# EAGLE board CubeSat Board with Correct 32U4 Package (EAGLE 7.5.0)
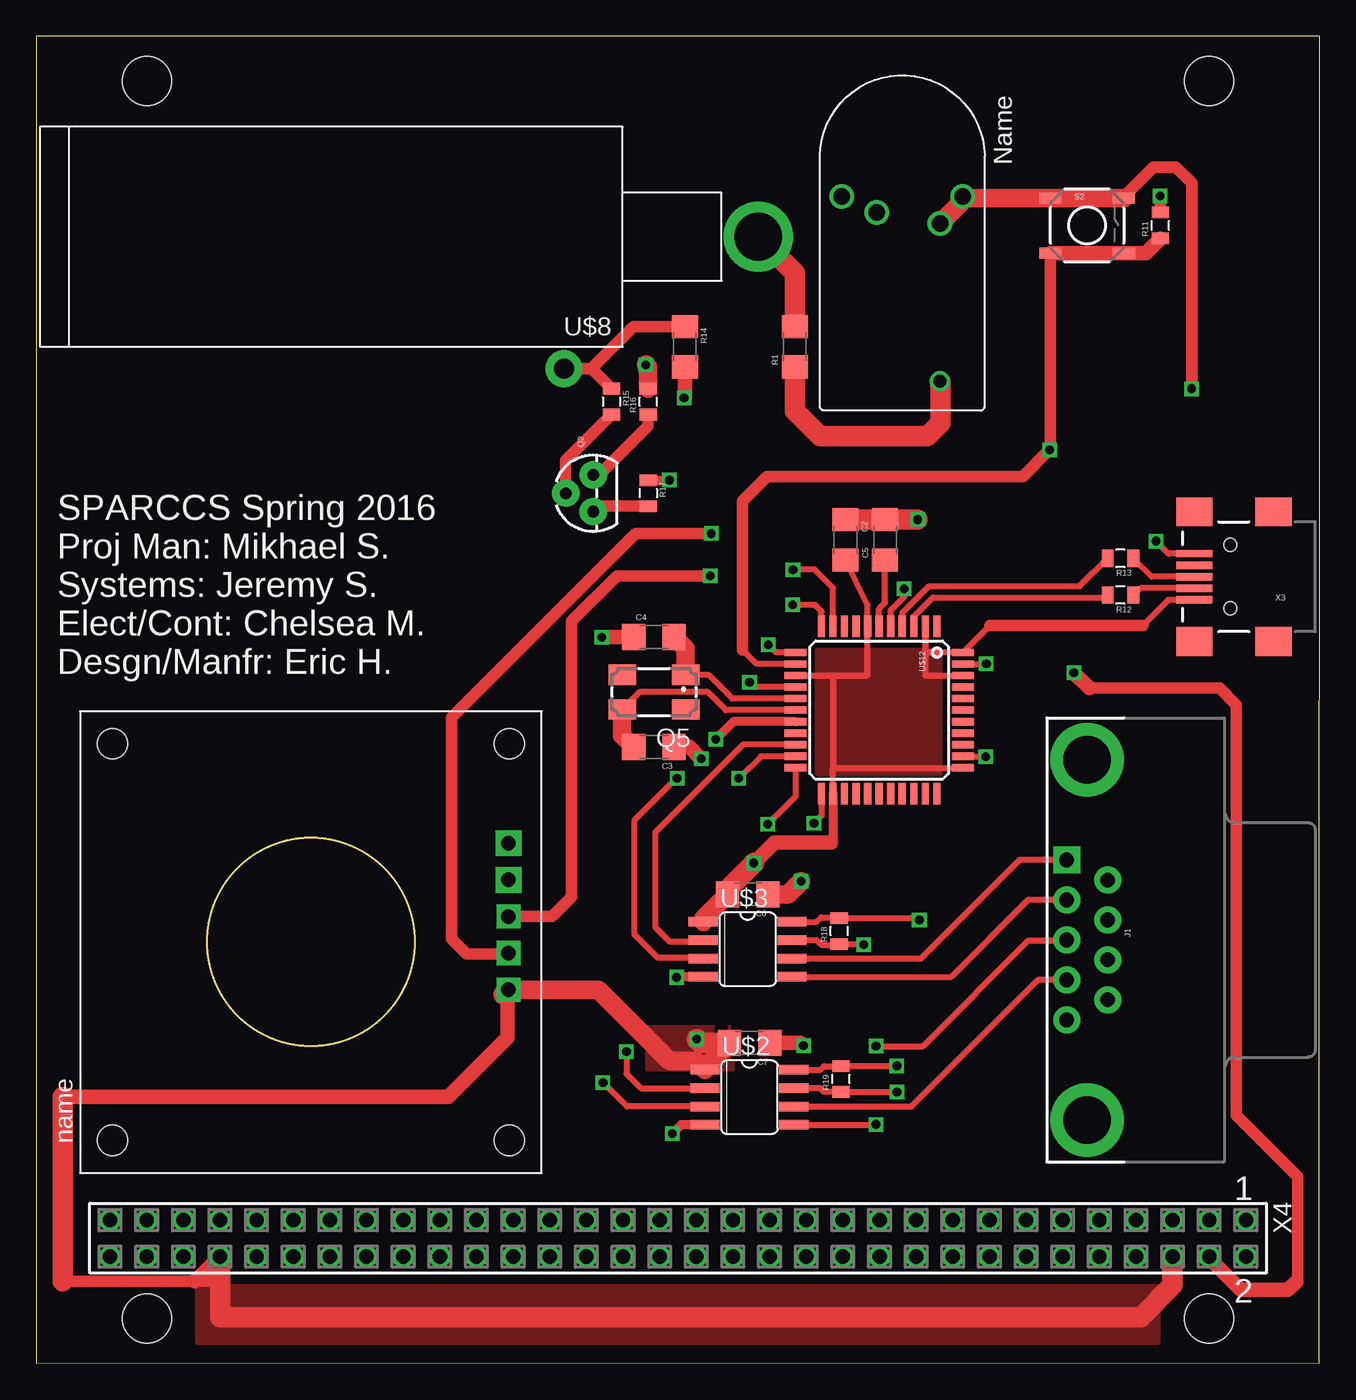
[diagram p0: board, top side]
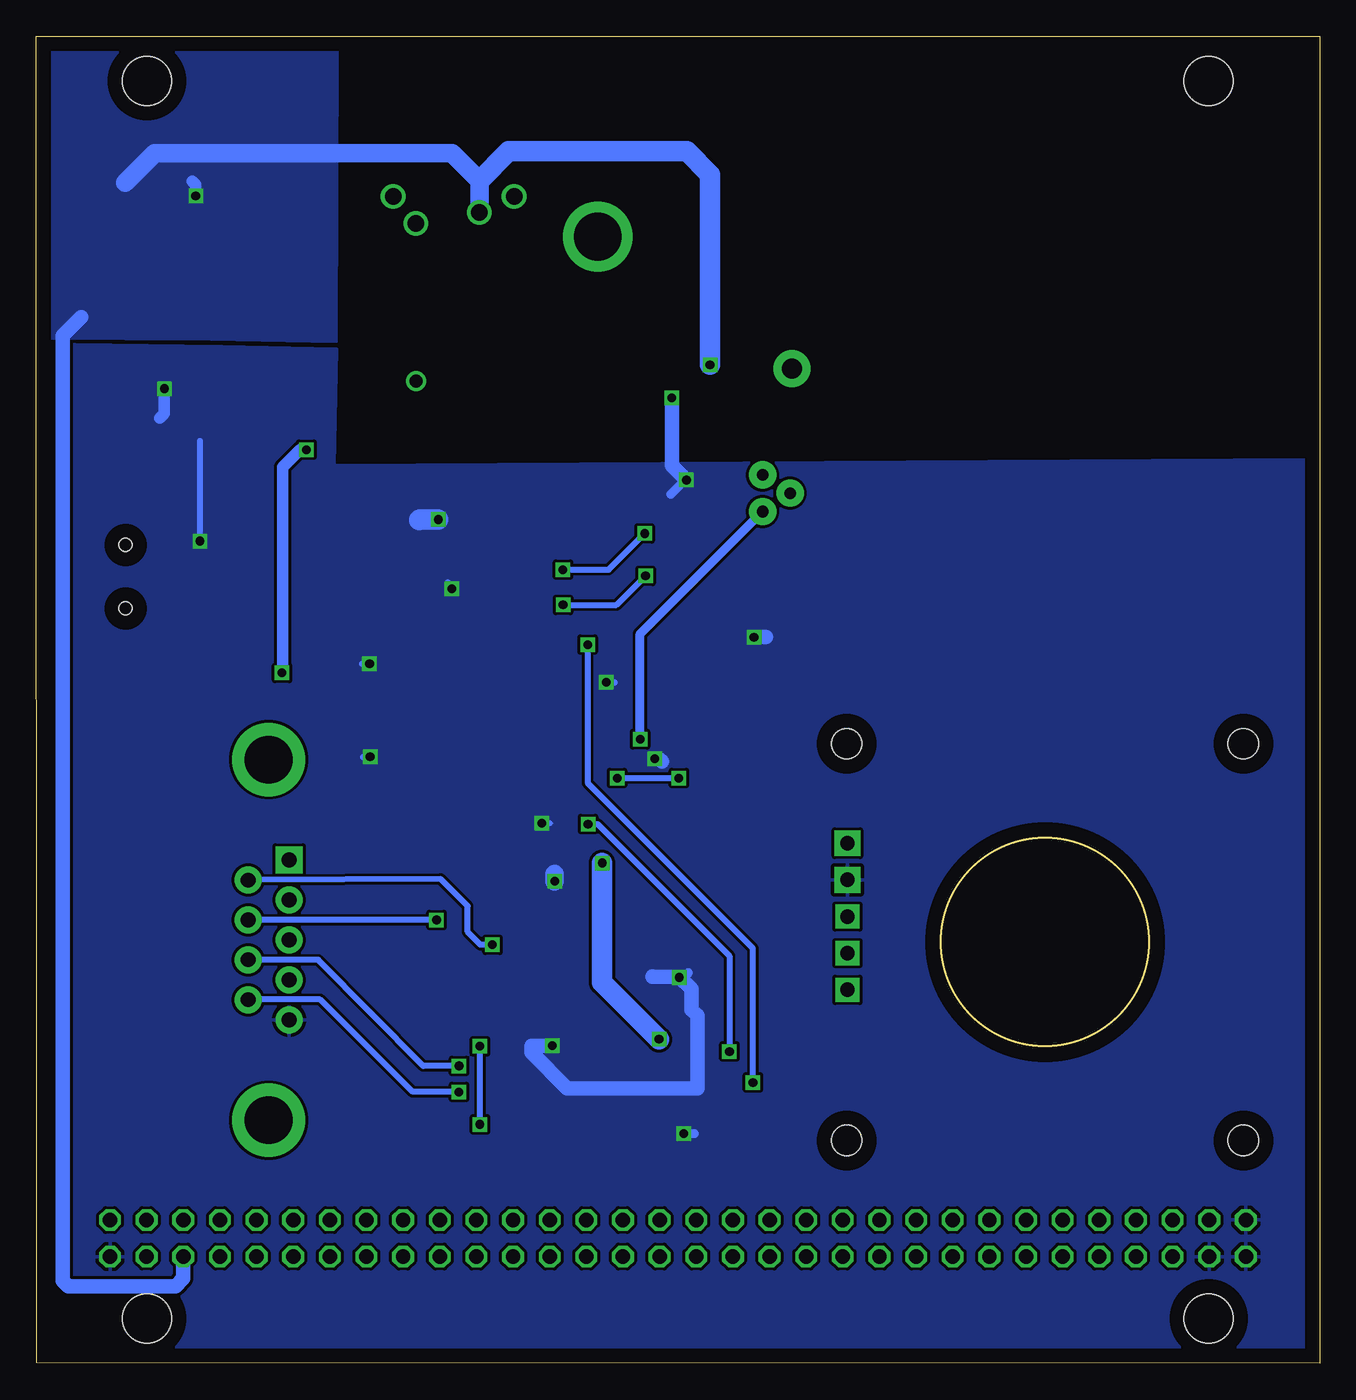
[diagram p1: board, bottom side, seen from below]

Size 89 x 92.02 mm. Coordinates in mm from the lower left corner, seen from the top.
Outline: 0,0 88.95,0.03 89,92.02 0,92.01 0,0
Copper layers (1*16): Top 0.035mm / dielectric 1.5mm / Bottom 0.035mm
Design rules "default": minimum track width 10mil, minimum drill 24mil, track to track 8mil, track to pad 8mil, pad to pad 8mil, via to via 8mil, smd to smd 8mil, copper to edge 40mil, drill to drill 8mil, minimum pad ring 10mil, minimum via ring 8mil, stop-mask expansion 4mil, vias tented up to drill 0mil, thermal gap 10mil
Holes 3.4 mm at 7.7,3.1 81.3,3.1 81.3,88.9 7.7,88.9

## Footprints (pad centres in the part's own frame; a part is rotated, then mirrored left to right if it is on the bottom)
1206 = smd 1.6 x 1.8: 1 -1.4,0; 2 1.4,0
ASERIES = drill 1.143: (+)IN -2.032,-1.778; (-)IN -3.15,4.191; CNTRL -3.15,-4.191; HVRTN -1.27,2.616 | drill 0.889: HVOUT 9.652,2.616
DB9 = drill 1.016 pad 1.88 square: 1 -5.54,-1.42 | drill 1.016 pad 1.88: 2 -2.77,-1.42; 3 0,-1.42; 4 2.77,-1.42; 5 5.54,-1.42; 6 -4.15,1.42; 7 -1.38,1.42; 8 1.38,1.42; 9 4.15,1.42 | drill 3.302 pad 5.08: G1 -12.5,0; G2 12.5,0
TO-92 = drill 0.813 pad 1.88: 1 -1.27,0; 2 0,1.905; 3 1.27,0
CTS406 = smd 1.9 x 1.4: 1 -2.2,-1.2; 2 2.2,-1.2; 3 2.2,1.2; 4 -2.2,1.2
0805 = smd 0.8 x 1.2: 1 -0.9,0; 2 0.9,0
TACTILE_SWITCH_SMD = smd 1.524 x 0.762: 1 -2.54,1.905; 2 2.54,1.905; 3 -2.54,-1.905; 4 2.54,-1.905
SO-08 = smd 0.66 x 2.032: 1 -1.905,-3.073; 2 -0.635,-3.073; 3 0.635,-3.073; 4 1.905,-3.073; 5 1.905,3.073; 6 0.635,3.073; 7 -0.635,3.073; 8 -1.905,3.073
GEIGER_TUBE = drill 1.4 pad 2.54: GND 13.462,9.144 | drill 3.302 pad 4.826: VCC 0,0
UCAM-II = drill 1 pad 1.676 square: 5V -3.31,-13.7; RX 1.77,-13.7; TX -0.77,-13.7 | drill 1 pad 1.778 square: GND 4.31,-13.7; RES 6.85,-13.7 | hole 2.1: -13.75,-13.75; 13.75,-13.75; 13.75,13.75; -13.75,13.75
SPARKFUN-DIGITALIC_TQFP44 = smd 1.5 x 0.5: 1 -5.8,4; 2 -5.8,3.2; 3 -5.8,2.4; 4 -5.8,1.6; 5 -5.8,0.8; 6 -5.8,0; 7 -5.8,-0.8; 8 -5.8,-1.6; 9 -5.8,-2.4; 10 -5.8,-3.2; 11 -5.8,-4; 23 5.8,-4; 24 5.8,-3.2; 25 5.8,-2.4; 26 5.8,-1.6; 27 5.8,-0.8; 28 5.8,0; 29 5.8,0.8; 30 5.8,1.6; 31 5.8,2.4; 32 5.8,3.2; 33 5.8,4 | smd 0.5 x 1.5: 12 -4,-5.8; 13 -3.2,-5.8; 14 -2.4,-5.8; 15 -1.6,-5.8; 16 -0.8,-5.8; 17 0,-5.8; 18 0.8,-5.8; 19 1.6,-5.8; 20 2.4,-5.8; 21 3.2,-5.8; 22 4,-5.8; 34 4,5.8; 35 3.2,5.8; 36 2.4,5.8; 37 1.6,5.8; 38 0.8,5.8; 39 0,5.8; 40 -0.8,5.8; 41 -1.6,5.8; 42 -2.4,5.8; 43 -3.2,5.8; 44 -4,5.8
USB-MINIB = smd 2.5 x 0.5: D+ 2.5,0; D- 2.5,0.8; GND 2.5,-1.6; ID 2.5,-0.8; VBUS 2.5,1.6 | smd 2.5 x 2: MTN1 -3,4.5; MTN2 2.5,4.5; MTN3 -3,-4.5; MTN4 2.5,-4.5 | hole 0.9: 0,2.2; 0,-2.2
SSW-132-02-S-D = drill 1 pad 1.5 octagon: 1 -39.37,-1.27; 2 -39.37,1.27; 3 -36.83,-1.27; 4 -36.83,1.27; 5 -34.29,-1.27; 6 -34.29,1.27; 7 -31.75,-1.27; 8 -31.75,1.27; 9 -29.21,-1.27; 10 -29.21,1.27; 11 -26.67,-1.27; 12 -26.67,1.27; 13 -24.13,-1.27; 14 -24.13,1.27; 15 -21.59,-1.27; 16 -21.59,1.27; 17 -19.05,-1.27; 18 -19.05,1.27; 19 -16.51,-1.27; 20 -16.51,1.27; 21 -13.97,-1.27; 22 -13.97,1.27; 23 -11.43,-1.27; 24 -11.43,1.27; 25 -8.89,-1.27; 26 -8.89,1.27; 27 -6.35,-1.27; 28 -6.35,1.27; 29 -3.81,-1.27; 30 -3.81,1.27; 31 -1.27,-1.27; 32 -1.27,1.27; 33 1.27,-1.27; 34 1.27,1.27; 35 3.81,-1.27; 36 3.81,1.27; 37 6.35,-1.27; 38 6.35,1.27; 39 8.89,-1.27; 40 8.89,1.27; 41 11.43,-1.27; 42 11.43,1.27; 43 13.97,-1.27; 44 13.97,1.27; 45 16.51,-1.27; 46 16.51,1.27; 47 19.05,-1.27; 48 19.05,1.27; 49 21.59,-1.27; 50 21.59,1.27; 51 24.13,-1.27; 52 24.13,1.27; 53 26.67,-1.27; 54 26.67,1.27; 55 29.21,-1.27; 56 29.21,1.27; 57 31.75,-1.27; 58 31.75,1.27; 59 34.29,-1.27; 60 34.29,1.27; 61 36.83,-1.27; 62 36.83,1.27; 63 39.37,-1.27; 64 39.37,1.27

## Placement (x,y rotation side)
C2  0.1uF  [1206]  56.11,57.09 270 top
C3  18pF  [1206]  42.84,42.73 180 top
C4  18pF  [1206]  42.84,50.35 0 top
C5  1uF  [1206]  58.85,57.09 90 top
C6  0.1uF  [1206]  49.33,32.52 180 top
C7  0.1uF  [1206]  49.47,22.23 180 top
DC-HVDC  A06  [ASERIES]  60.05,77.75 270 top
J1  DB9 Connector  [DB9]  72.87,29.36 270 top
Q2  MPSA18  [TO-92]  38.62,60.33 90 top
Q5  16MHz  [CTS406]  42.84,46.54 180 top
R1  10M  [1206]  52.59,70.48 90 top
R11  10k  [0805]  77.94,78.89 90 top
R12  22  [0805]  75.17,53.27 180 top
R13  22  [0805]  75.17,55.8 180 top
R14  1M  [1206]  44.98,70.48 270 top
R15  10M  [0805]  39.9,66.67 270 top
R16  15k  [0805]  42.44,66.67 90 top
R17  1M  [0805]  42.44,60.33 270 top
R18  120  [0805]  55.68,29.98 90 top
R19  120  [0805]  55.8,19.73 90 top
S2  Reset  [TACTILE_SWITCH_SMD]  72.86,78.89 0 top
U$2  MAX488  [SO-08]  49.45,18.45 270 top
U$3  MAX488  [SO-08]  49.33,28.71 270 top
U$8  GEIGER_TUBELND712  [GEIGER_TUBE]  50.05,78.11 180 top
U$9  UCAM-II  [UCAM-II]  19.05,29.21 90 top
U$12  ATMEGA32U4TQFP  [SPARKFUN-DIGITALIC_TQFP44]  58.45,45.29 270 top
X3  USBSMD  [USB-MINIB]  82.78,54.53 180 top
X4  SSW-132-02-S-D  [SSW-132-02-S-D]  44.5,8.68 180 top

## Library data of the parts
C2-C7 = SparkFun-Passives
DC-HVDC = aseries
J1 = SparkFun-Connectors; PROD_ID: CONN-08194
Q2 R1 R11-R19 S2 U$8 X3 = SparkFun
Q5 = crystal; OC_FARNELL: unknown; OC_NEWARK: unknown
U$2 U$3 = max
U$9 = camera
U$12 = SparkFun-Retired; PROD_ID: IC-11161
X4 = con-samtec; MPN: SSW-132-02-S-D; OC_FARNELL: unknown; OC_NEWARK: 11P9837

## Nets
CTS+: J1.9 R19.1 U$2.7
CTS-: J1.8 R19.2 U$2.8
GND: C2.1 C3.1 C4.1 C5.2 C6.1 C7.1 DC-HVDC.(-)IN DC-HVDC.HVRTN J1.5 R14.2 R17.1 S2.1 S2.2 U$2.4 U$3.4 U$9.GND U$12.5 U$12.15 U$12.23 U$12.35 U$12.43 X3.GND X4.2 X4.62 X4.63 X4.64
MISO: U$9.RX U$12.11
MOSI: U$9.TX U$12.10
N$1: C3.2 Q5.3 U$12.17
N$2: R1.2 U$8.VCC
N$3: R14.1 R15.1 U$8.GND
N$4: DC-HVDC.HVOUT R1.1
N$5: Q2.2 R15.2
N$7: C4.2 Q5.1 U$12.16
N$8: Q2.3 R16.1
N$19: R12.1 X3.D-
N$21: R13.1 X3.D+
N$24: R12.2 U$12.3
N$25: R13.2 U$12.4
N$26: C5.1 U$12.6
OUT: Q2.1 R17.2 U$12.18
RST: R11.1 S2.3 S2.4 U$12.13 X4.4
RTS+: J1.4 U$2.6
RTS-: J1.3 U$2.5
RX: U$3.2 U$12.20
RX+: J1.7 R18.2 U$3.8
RX-: J1.6 R18.1 U$3.7
TX: U$3.3 U$12.21
TX+: J1.2 U$3.5
TX-: J1.1 U$3.6
VCC: C2.2 C6.2 C7.2 DC-HVDC.(+)IN R11.2 R16.2 U$2.1 U$3.1 U$9.5V U$12.2 U$12.7 U$12.14 U$12.24 U$12.34 U$12.42 U$12.44 X3.VBUS X4.6 X4.58
~CTS: U$2.2 U$12.22
~RTS: U$2.3 U$12.12

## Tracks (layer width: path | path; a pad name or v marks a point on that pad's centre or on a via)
CTS+  (via drill 0.6)
  Top 0.406: U$2.7 54.35,19.09 54.59,18.85 55.77,18.85 R19.1 59.34,18.82 v59.68,18.82
  Bottom 0.406: v59.68,18.82 62.88,18.83 69.31,25.23 74.27,25.23 J1.9
CTS-  (via drill 0.6)
  Top 0.406: U$2.8 54.37,20.36 54.62,20.61 55.78,20.61 R19.2 v59.67,20.62
  Bottom 0.406: v59.67,20.62 62.16,20.62 69.43,27.98 74.21,27.98 J1.8
GND  (via drill 0.6)
  Top 0.406: U$12.15 49.77,46.89 v49.45,47.21 | U$12.5 59.24,52.23 60.18,53.17 v60.18,53.7 | U$12.43 v65.87,48.49 v65.88,48.49 | U$12.35 65.81,42.09 v65.83,42.06 | U$12.23 54.45,37.98 v53.92,37.45 | X3.GND 78.5,56.13 v77.64,57.01
  Top 0.61: U$2.4 44.72,16.55 v44.1,15.94 | R17.1 43.9,61.23 v43.91,61.24 | U$3.4 44.45,26.8 v44.4,26.76
  Top 0.813: S2.2 75.39,80.89 77.44,82.94 79,82.94 80.11,81.84 v80.11,67.58
  Top 1.016: C3.1 45.29,42.73 v46.1,41.91 | C4.1 v39.23,50.35 | R14.2 44.98,66.99 v44.92,66.94 | C7.1 53.01,22.23 v53.2,22.03
  Top 1.27: C6.1 52.14,32.52 v53.04,33.42 | S2.2 S2.1 64.35,80.79 DC-HVDC.(-)IN 64.24,80.59 DC-HVDC.HVRTN
  Top 1.422: C2.1 C5.2 v61.1,58.49 v61.11,58.5
  Bottom 0.406: v49.45,47.21 49.05,47.21 49.04,47.22 48.91,47.22 48.9,47.2 48.88,47.22 | v60.18,53.7 60.18,53.88 60.47,54.16 | v65.88,48.49 66.29,48.49 66.3,48.48 66.3,48.49 66.42,48.49 66.42,48.5 | v65.83,42.06 66.31,42.06 66.33,42.04 | v53.92,37.45 53.38,37.45 53.37,37.45 | v77.64,57.01 77.64,63.95
  Bottom 0.61: v44.1,15.94 43.36,15.94 | v43.91,61.24 43.99,61.24 44.98,60.26 | v44.4,26.76 44.09,26.76 43.77,27.08
  Bottom 0.813: v80.11,67.58 80.11,65.85 80.42,65.53
  Bottom 1.016: v46.1,41.91 45.8,41.91 45.61,41.73 | v39.23,50.35 38.38,50.35 | v44.92,66.94 44.92,62.25 v43.91,61.24 | v53.2,22.03 54.65,22.03 54.66,22.02 54.66,21.55 52.17,19.07 43.15,19.07 43.15,24.11 43.55,24.52 43.55,25.95 44.41,26.8 U$3.4 46.27,26.81 46.27,26.82 46.26,26.84 U$3.4 46.24,26.78
  Bottom 1.27: v53.04,33.42 53.04,33.94
  Bottom 1.422: v61.11,58.5 62.42,58.5 62.45,58.47
  pour Bottom: 0.16,0.15 88.81,0.21 88.78,70.64 76.19,70.5 76.11,70.48 68.14,70.31 68.33,62.23 0.35,62.64 0.14,6.32
MISO  (via drill 0.6)
  Top 0.406: U$12.11 54.45,52.12 53.98,52.58 v52.46,52.58 | U$9.RX
  Top 0.813: v46.74,54.59 40.27,54.59 37.13,51.46 37.13,32.35 35.77,30.98 U$9.RX
  Bottom 0.406: v52.46,52.58 48.76,52.58 v46.74,54.59
MOSI  (via drill 0.6)
  Top 0.406: U$12.10 55.24,53.74 53.95,55.04 52.48,55.04 v52.47,55.02
  Top 0.813: v46.8,57.53 41.56,57.53 28.8,44.77 28.8,29.41 29.83,28.39 32.7,28.39 U$9.TX
  Bottom 0.406: v52.47,55.02 49.3,55.02 v46.8,57.53
N$1
  Top 0.406: U$12.17 47.82,45.29 46.58,46.53 41.83,46.53 Q5.3
  Top 1.27: Q5.3 40.63,43.53 C3.2
N$2
  Top 1.422: R1.2 52.59,75.56 U$8.VCC
N$3
  Top 0.813: R15.1 38.51,68.96 | 38.51,68.96 U$8.GND | R14.1 41.43,71.89 38.51,68.96
N$4
  Top 1.422: R1.1 52.59,66.03 54.33,64.3 61.79,64.3 62.69,65.19 62.69,68.07 DC-HVDC.HVOUT
N$5
  Top 0.813: Q2.2 36.72,62.6 R15.2
N$7
  Top 0.406: U$12.16 48.27,46.09 46.65,47.71 45.06,47.71 Q5.1
  Top 1.27: C4.2 45.03,49.55 Q5.1
N$8
  Top 0.813: Q2.3 39.04,61.59 42.44,64.99 R16.1
N$19
  Top 0.406: X3.D- 76.53,53.73 R12.1
N$21
  Top 0.406: X3.D+ 77.33,54.53 R13.1
N$24
  Top 0.406: U$12.3 60.84,51.78 62.17,53.11 74.11,53.11 R12.2
N$25
  Top 0.406: U$12.4 60.05,52.05 61.88,53.88 72.34,53.88 R13.2
N$26
  Top 0.406: U$12.6 58.45,52.33 58.86,52.74 C5.1
  Top 1.016: 58.84,55.69 C5.1
OUT  (via drill 0.6)
  Top 0.61: U$12.18 48.34,44.49 v47.12,43.27
  Top 0.813: R17.2 38.99,59.42 Q2.1
  Bottom 0.61: v47.12,43.27 47.12,50.56 Q2.1
RST  (via drill 0.6)
  Top 0.406: U$12.13 49.95,48.49 48.98,49.47
  Top 0.813: 48.98,49.47 48.98,59.78 50.68,61.48 68.4,61.48 v70.25,63.34 70.31,63.4 S2.3 | 73,46.81 82.06,46.81 83.21,45.66 83.21,17.2 87.47,12.94 87.47,5.79 87.36,5.67
  Top 1.016: S2.3 S2.4 76.93,76.98 R11.1 | X4.4 81.33,7.28 83.52,5.09 86.77,5.09 87.36,5.67 | 73,46.81 v71.94,47.87
  Bottom 0.813: v70.25,63.34 70.7,63.34 71.9,62.13 71.9,47.91 v71.94,47.87
RTS+
  Top 0.406: U$2.6 60.7,17.82 69.48,26.61 71.44,26.61 J1.4
RTS-  (via drill 0.6)
  Top 0.406: U$2.5 58.2,16.55 v58.23,16.57 | v58.23,21.98 61.48,21.98 68.81,29.32 71.41,29.32 J1.3
  Bottom 0.406: v58.23,16.57 v58.23,21.98
RX
  Top 0.406: U$12.20 48.99,42.89 42.91,36.81 42.91,30.26 43.91,29.25 46.17,29.25 U$3.2
RX+  (via drill 0.6)
  Top 0.406: U$3.8 54.12,30.61 54.44,30.93 55.62,30.93 R18.2 61.22,30.88 v61.23,30.74
  Bottom 0.406: v61.23,30.74 J1.7
RX-  (via drill 0.6)
  Top 0.406: U$3.7 54.1,29.34 54.44,29.02 55.62,29.02 R18.1 57.31,29.08 v57.37,29.02
  Bottom 0.406: v57.37,29.02 58.19,29.02 59.08,29.92 59.08,31.71 60.95,33.58 74.22,33.52 J1.6
TX  (via drill 0.6)
  Top 0.406: U$12.21 50.23,42.09 v48.72,40.57 | v44.44,40.57 44.4,40.57 41.46,37.63 41.46,29.77 43.09,28.14 46.19,28.14 U$3.3
  Bottom 0.406: v48.72,40.57 v44.44,40.57
TX+
  Top 0.406: U$3.5 63.45,26.8 68.81,32.16 71.42,32.16 J1.2
TX-
  Top 0.406: U$3.6 61.35,28.07 68.2,34.92 71.42,34.92 J1.1
VCC  (via drill 0.6)
  Top 0.406: C2.2 57.65,52.58 U$12.7 57.65,47.69 55.24,47.69 | X3.VBUS 78.49,52.94 76.72,51.16 | U$12.42 61.65,47.69 U$12.2 61.65,49.29 U$12.44 66.12,51.16 | U$12.24 55.24,41.29 | 55.24,41.29 U$12.34 | U$12.14 55.24,47.69 | 55.24,47.69 55.24,41.29
  Top 0.61: U$12.24 55.24,36.27 55.09,36.11
  Top 0.813: 76.72,51.16 66.12,51.16 | R11.2 77.94,80.92 v77.92,80.94 | 12.63,5.7 1.86,5.7
  Top 1.016: X4.58 10.99,5.7 | 55.09,36.11 51.17,36.11 v49.76,34.69 | 1.86,18.47 28.57,18.47 32.69,22.59 32.69,25.84 U$9.5V
  Top 1.27: U$3.1 46.26,30.85 C6.2 | C7.2 46.38,20.54 U$2.1 45.75,20.99 43.91,20.99 38.99,25.9 U$9.5V | R16.2 42.44,69.06 v42.27,69.22 | 12.63,5.7 12.75,5.58
  Top 1.422: X4.58 12.75,5.58 12.75,3.21 76.59,3.21 78.78,5.41 78.78,7.45 X4.6 | 1.86,5.7 1.86,18.47 | 32.42,25.57 U$9.5V | C7.2 46.06,22.23 v45.81,22.48 | v49.76,34.69 47.93,32.87 C6.2
  Bottom 0.813: v77.92,80.94 77.92,81.71 78.18,81.97
  Bottom 1.016: 85.86,72.53 87.15,71.24 87.15,5.74 86.77,5.36 79.31,5.36 78.78,5.89 78.78,7.45 X4.6
  Bottom 1.27: DC-HVDC.(+)IN 58.27,82 60.16,83.89 80.75,83.89 82.81,81.83
  Bottom 1.422: v45.81,22.48 49.76,26.43 v49.76,34.69 | v42.27,69.22 42.27,82.41 43.88,84.02 56.24,84.02 58.27,82
  pour Top: 54.23,49.42 62.63,49.42 62.63,40.91 54.19,40.91 54.19,49.42
  pour Top: 11.21,1.49 77.76,1.49 77.76,5.29 11.21,5.29 11.21,1.48
  pour Top: 42.39,20.36 48.3,20.36 48.3,23.34 42.35,23.34 42.35,20.36
  pour Bottom: 76.84,71.02 88.78,71.06 88.74,91.76 68.13,91.63 68.19,70.85
~CTS  (via drill 0.6)
  Top 0.406: U$12.22 52.65,39.3 v50.73,37.39 | v40.93,21.62 40.93,20.07 41.94,19.07 46.36,19.07 U$2.2
  Bottom 0.406: v50.73,37.39 50.06,37.39 40.93,28.25 v40.93,21.62
~RTS  (via drill 0.6)
  Top 0.406: U$12.12 51.29,49.29 v50.76,49.82 | U$2.3 40.95,17.82 v39.3,19.47
  Bottom 0.406: v50.76,49.82 50.76,40.24 39.3,28.79 v39.3,19.47

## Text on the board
tNames: SPARCCS Spring 2016 / Proj Man: Mikhael S. / Systems: Jeremy S. / Elect/Cont: Chelsea M. / Desgn/Manfr: Eric H.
